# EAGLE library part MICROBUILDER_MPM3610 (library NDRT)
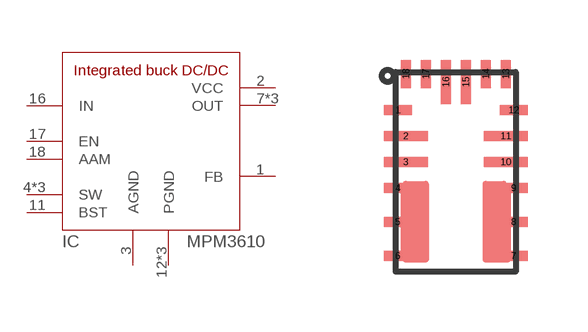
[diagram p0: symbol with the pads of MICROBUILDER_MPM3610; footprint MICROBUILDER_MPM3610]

Designator prefix IC

## MICROBUILDER_MPM3610  [MICROBUILDER_MPM3610]
1  FB  in
2  VCC  pwr
3  AGND  pwr
4  SW  pas
5  SW  pas
6  SW  pas
7  OUT  sup
8  OUT  sup
9  OUT  sup
11  BST  pas
12  PGND  pwr
13  PGND  pwr
14  PGND  pwr
16  IN  pwr
17  EN  in
18  AAM  in

## Footprint MICROBUILDER_MPM3610 (pad centres in mm)
smd 0.7 x 0.25: 1 -1.45,1.55; 4 -1.45,-0.4; 5 -1.45,-1.25; 6 -1.45,-2.1; 7 1.45,-2.1; 8 1.45,-1.25; 9 1.45,-0.4; 12 1.45,1.55
smd 1.1 x 0.25: 2 -1.25,0.9; 3 -1.25,0.25; 10 1.25,0.25; 11 1.25,0.9
smd 0.25 x 0.7: 13 1.25,2.45; 14 0.75,2.45; 17 -0.75,2.45; 18 -1.25,2.45
smd 0.25 x 1.1: 15 0.25,2.25; 16 -0.25,2.25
